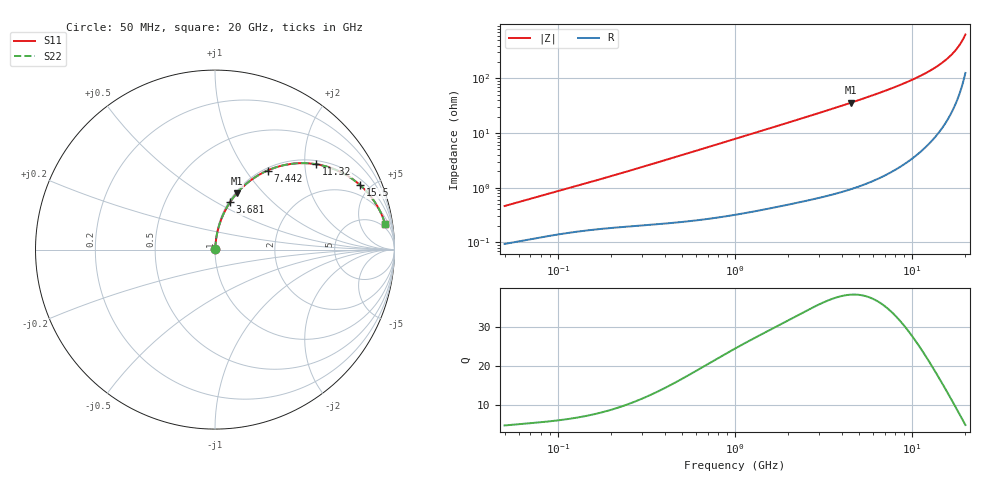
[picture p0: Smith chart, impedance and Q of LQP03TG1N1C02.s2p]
!Murata Part Number: LQP03TG1N1C02
!These Parameters are Measured in Series Mode Connection
!  o--[Z]--o
!Port1  Port2
!  o-------o
!Freq. Start=50[MHz] Stop=20[GHz], 401[Steps]
# Hz S RI R 50
!Freq.(Hz) S11(Real) S11(Imag) S21(Real) S21(Imag) S12(Real) S12(Imag) S22(Real) S22(Imag)
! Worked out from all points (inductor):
!   401 points, 50 MHz to 20 GHz, reference 50 ohm
!   read as one part in series: L = 1.41 nH near 51.52 MHz
!   highest Q = 38.3 at 4.54 GHz (marker M1), where L = 1.27 nH
!   S11 on the Smith chart (normalised r, x): 50 MHz: 1.00, +0.01; 3.681 GHz: 1.02, +0.58; 7.442 GHz: 1.04, +1.27; 11.32 GHz: 1.09, +2.28; 15.5 GHz: 1.31, +4.35; 20 GHz: 4, +12
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5e7  0.000954 0.00451  0.999 -0.00451  0.999 -0.00451  0.000954 0.00451
1.364002e8  0.00173 0.0113  0.9983 -0.0113  0.9983 -0.0113  0.00173 0.0113
3.721004e8  0.00301 0.0293  0.997 -0.0293  0.997 -0.0293  0.00301 0.0293
6.380365e8  0.00505 0.0497  0.995 -0.0497  0.995 -0.0497  0.00505 0.0497
1e9  0.00916 0.077  0.9908 -0.077  0.9908 -0.077  0.00916 0.077
1.714689e9  0.0216 0.1297  0.9784 -0.1297  0.9784 -0.1297  0.0216 0.1297
2.728004e9  0.0485 0.2009  0.9515 -0.2009  0.9515 -0.2009  0.0485 0.2009
3.680849e9  0.0831 0.2631  0.9169 -0.2631  0.9169 -0.2631  0.0831 0.2631
4.539627e9  0.1217 0.3141  0.8783 -0.3141  0.8783 -0.3141  0.1217 0.3141
5.856089e9  0.1925 0.3812  0.8075 -0.3812  0.8075 -0.3812  0.1925 0.3812
7.442007e9  0.2926 0.4406  0.7074 -0.4406  0.7074 -0.4406  0.2926 0.4406
9.316812e9  0.4227 0.4774  0.5773 -0.4774  0.5773 -0.4774  0.4227 0.4774
1.131968e10  0.5634 0.4757  0.4366 -0.4757  0.4366 -0.4757  0.5634 0.4757
1.238412e10  0.6343 0.4589  0.3657 -0.4589  0.3657 -0.4589  0.6343 0.4589
1.334722e10  0.6943 0.4352  0.3057 -0.4352  0.3057 -0.4352  0.6943 0.4352
1.438523e10  0.7534 0.4018  0.2466 -0.4018  0.2466 -0.4018  0.7534 0.4018
1.550395e10  0.8097 0.3585  0.1903 -0.3585  0.1903 -0.3585  0.8097 0.3585
1.670968e10  0.8608 0.3051  0.1392 -0.3051  0.1392 -0.3051  0.8608 0.3051
1.774144e10  0.8964 0.2556  0.1036 -0.2556  0.1036 -0.2556  0.8964 0.2556
1.855685e10  0.9192 0.215  0.0808 -0.215  0.0808 -0.215  0.9192 0.215
1.940974e10  0.9383 0.1717  0.0617 -0.1717  0.0617 -0.1717  0.9383 0.1717
2e10  0.9487 0.1416  0.0513 -0.1416  0.0513 -0.1416  0.9487 0.1416
